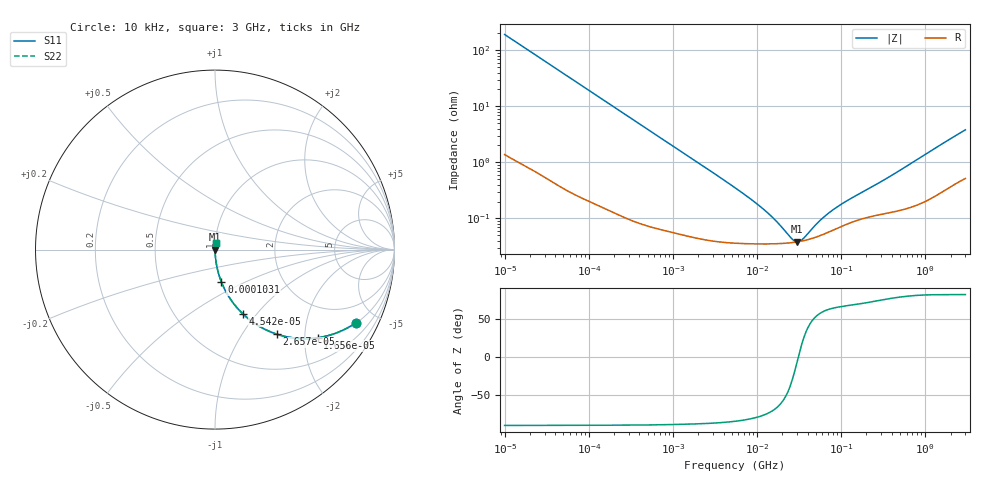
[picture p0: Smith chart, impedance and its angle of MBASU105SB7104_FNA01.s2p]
! MBASU105SB7104_FNA01  S-PARAMETER MODEL  ( Standard Model )
! Model Generated by TAIYO YUDEN Corporation (http://www.ty-top.com)
! Version 2.0
! TAIYO YUDEN Control No. 230906
! Copyright(c) 2014 TAIYO YUDEN CO.,LTD. All Rights Reserved.
! Product Description (link to TY-COMPAS)
! https://ds.yuden.co.jp/TYCOMPAS/or/detail?pn=MBASU105SB7104KFNA01&u=M
! Products Name : Multilayer Ceramic Capacitors
! Characteristics :
!  Capacitance : 0.1 [uF] , Rated Voltage : 50 [V] , TCC : X7R
!  Case Size : 1.0 x 0.5 / 0.039 x 0.02 [mm/inch] , Thickness : 0.5 / 0.02 [mm/inch]
!  (Conditions: Temperature = 25 [degC] , DC Bias Voltage = 0 [V])
! External Node Assignments :
!  1  o---| |---o  2
! GND o---------o GND
! Frequency Range : 10kHz  -  3GHz  [ 401 STEP ]
# MHZ S RI R 50
! Freq[MHz].  S11 Real  S11 Imag  S21 Real  S21 Imag  S12 Real  S12 Imag  S22 Real  S22 Imag
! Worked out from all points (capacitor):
!   401 points, 10 kHz to 3 GHz, reference 50 ohm
!   read as one part in series: C = 83.3 nF near 10.65 kHz
!   lowest |Z| = 38.3 mohm at 30.06 MHz (marker M1)
!   series resonance near 30.95 MHz, so ESL is about 320 pH
!   S11 on the Smith chart (normalised r, x): 10 kHz: 1.03, -3.82; 16.56 kHz: 1.02, -2.31; 26.57 kHz: 1.01, -1.44; 45.42 kHz: 1.01, -0.85; 103.1 kHz: 1.00, -0.37; 3 GHz: 1.01, +0.08
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0.01  0.7831 -0.4086  0.2169 0.4086  0.2169 0.4086  0.7831 -0.4086
0.012083  0.713 -0.4487  0.287 0.4487  0.287 0.4487  0.713 -0.4487
0.016561  0.5712 -0.491  0.4288 0.491  0.4288 0.491  0.5712 -0.491
0.020651  0.4628 -0.4946  0.5372 0.4946  0.5372 0.4946  0.4628 -0.4946
0.026575  0.3438 -0.4708  0.6562 0.4708  0.6562 0.4708  0.3438 -0.4708
0.035295  0.2305 -0.4169  0.7695 0.4169  0.7695 0.4169  0.2305 -0.4169
0.045421  0.1542 -0.3568  0.8458 0.3568  0.8458 0.3568  0.1542 -0.3568
0.082683  0.0536 -0.2203  0.9464 0.2203  0.9464 0.2203  0.0536 -0.2203
0.103102  0.0357 -0.1803  0.9643 0.1803  0.9643 0.1803  0.0357 -0.1803
0.234035  0.00793 -0.0822  0.9921 0.0822  0.9921 0.0822  0.00793 -0.0822
0.683653  0.00145 -0.0285  0.9985 0.0285  0.9985 0.0285  0.00145 -0.0285
5.477226  0.000373 -0.0035  0.9996 0.0035  0.9996 0.0035  0.000373 -0.0035
12.43293  0.000352 -0.00134  0.9996 0.00134  0.9996 0.00134  0.000352 -0.00134
17.04125  0.000354 -0.000812  0.9996 0.000812  0.9996 0.000812  0.000354 -0.000812
25.67485  0.000369 -0.00024  0.9996 0.00024  0.9996 0.00024  0.000369 -0.00024
30.05882  0.000381 -3.72e-05  0.9996 3.72e-05  0.9996 3.72e-05  0.000381 -3.72e-05
35.19136  0.000398 0.000163  0.9996 -0.000163  0.9996 -0.000163  0.000398 0.000163
45.28751  0.00044 0.000487  0.9996 -0.000487  0.9996 -0.000487  0.00044 0.000487
62.07353  0.000523 0.000911  0.9995 -0.000911  0.9995 -0.000911  0.000523 0.000911
90.61918  0.00067 0.00147  0.9993 -0.00147  0.9993 -0.00147  0.00067 0.00147
374.4521  0.00129 0.00537  0.9987 -0.00537  0.9987 -0.00537  0.00129 0.00537
3000  0.00652 0.0372  0.9935 -0.0372  0.9935 -0.0372  0.00652 0.0372
